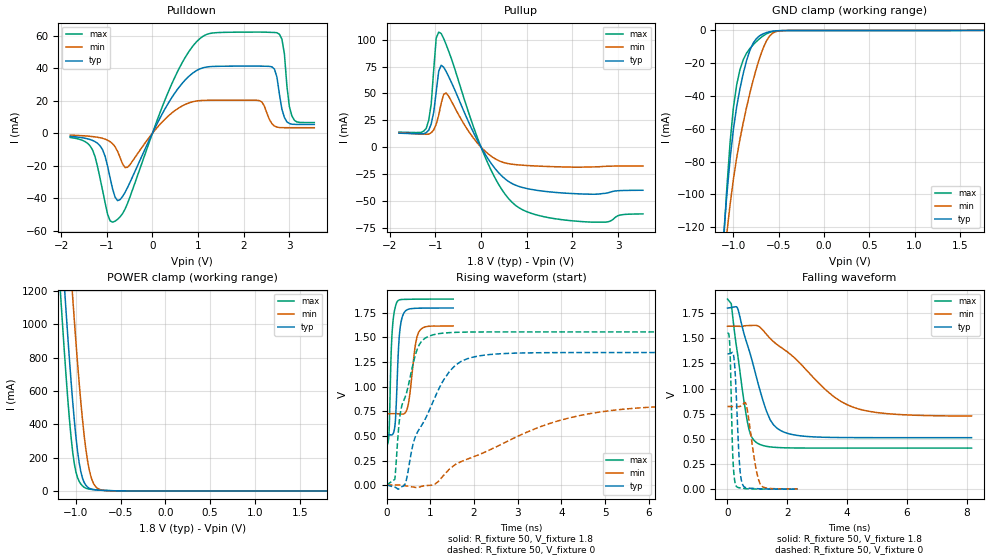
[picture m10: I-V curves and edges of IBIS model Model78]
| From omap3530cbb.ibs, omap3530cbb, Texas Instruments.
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| Model based on original model for BQ0234CS_7LM
|   Sub model BQ0234CS_7LM_PU_ON_1P8
[model]   Model78
|[Input Load]   PU
|[Output Drive]
|Voltage   1.8V
|Mode   I/O
Model_type   I/O
Polarity   Non-Inverting
Enable   Active-Low
Vinl =  0.63
Vinh =  1.17
Cref =  15.0000pF
Rref =  100.0000M
Vref =  0V
Vmeas =  0.9
C_comp   0.8818576p   0.7571797p   1.039848p
[Model Spec]
Vinl   0.63   0.567   0.6615
Vinh   1.17   1.053   1.2285
[Temperature Range]   25   125   -40
[Voltage Range]   1.8   1.62   1.89
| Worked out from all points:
|   slope of the pulldown table from 0 to 0.27 V, typ, clamps not added: 18.2 ohm
|   slope of the pullup table from 0 to 0.27 V, typ, clamps not added: 15.1 ohm
|   GND clamp passes 1 mA (typ) near -0.61 V on its own axis
|   POWER clamp passes 1 mA (typ) near -0.57 V on its own axis
|   rising waveform, R_fixture 50, V_fixture 1.8: 20-80 % time 81.1ps typ, 139ps min, 64.6ps max; typ from 0.513 V to 1.8 V
|   rising waveform, R_fixture 50, V_fixture 0: 20-80 % time 778ps typ, 2.51ns min, 382ps max; typ from 0.001 V to 1.35 V
|   falling waveform, R_fixture 50, V_fixture 1.8: 20-80 % time 757ps typ, 1.98ns min, 422ps max; typ from 1.8 V to 0.513 V
|   falling waveform, R_fixture 50, V_fixture 0: 20-80 % time 126ps typ, 250ps min, 81.5ps max; typ from 1.35 V to 0.002 V
[POWER_clamp]
-1.8V     7.03A      7.477A     6.772A
-1.182V   1.672A     2.34A      1.267A
-1.164V   1.518A     2.189A     1.114A
-1.127V   1.216A     1.889A     820.5mA
-1.073V   791.2mA    1.448A     431.2mA
-1.036V   538.2mA    1.164A     234.6mA
-963.6mV  169mA      647.7mA    57.34mA
-909.1mV  52.04mA    338.7mA    22.18mA
-872.7mV  24.24mA    189.9mA    13.43mA
-818.2mV  9.923mA    62.63mA    8.573mA
-709.1mV  3.896mA    5.034mA    3.819mA
1.8V      4.52nA     3.063nA    7.567nA
[Pulldown]
-1.8V     -1.896mA   -1.14mA    -2.549mA
-1.364V   -3.858mA   -1.868mA   -7.811mA
-1.145V   -7.758mA   -2.749mA   -27.9mA
-818.2mV  -39.37mA   -8.281mA   -54.21mA
-545.5mV  -33.5mA    -20.95mA   -43.25mA
654.5mV   30.89mA    16.9mA     43.69mA
1.418V    41.32mA    20.41mA    62.11mA
2.345V    41.43mA    20.12mA    62.44mA
2.618V    40.99mA    5.968mA    62.24mA
2.782V    24.07mA    3.525mA    61.09mA
3.055V    5.586mA    3.449mA    10.68mA
3.545V    5.467mA    3.446mA    6.63mA
[Pullup]
-1.8V     13mA       13.47mA    13.94mA
-1.2V     13.58mA    11.97mA    17.52mA
-1.091V   21.69mA    13.4mA     40.45mA
-1.036V   32.56mA    16.02mA    72.07mA
-981.8mV  51.55mA    21.35mA    101.5mA
-927.3mV  70.65mA    29.73mA    107.1mA
-818.2mV  74.4mA     49.19mA    101mA
-763.6mV  70.3mA     50.34mA    95.36mA
54.55mV   -4.056mA   -2.362mA   -5.695mA
709.1mV   -34.52mA   -16.04mA   -52.48mA
2.127V    -43.43mA   -18.65mA   -69.01mA
3.545V    -40.12mA   -17.52mA   -62.13mA
[GND_clamp]
-1.8V     -750.7mA   -623.3mA   -941.3mA
-1.109V   -125.7mA   -143.5mA   -129.9mA
-1.073V   -100.4mA   -123.9mA   -96.49mA
-1.036V   -78.3mA    -106.2mA   -68.25mA
-1V       -60.36mA   -90.76mA   -47.12mA
-963.6mV  -46.51mA   -77.61mA   -33.16mA
-890.9mV  -26.17mA   -56.18mA   -17.83mA
-818.2mV  -12.2mA    -38.34mA   -11.05mA
-709.1mV  -3.258mA   -16.62mA   -4.997mA
-600mV    -826.6uA   -3.389mA   -1.229mA
-490.9mV  -188uA     -312.2uA   -227.9uA
1.764V    -5.54uA    14.06uA    -26.2uA
[Ramp]
dV/dt_f  0.7805925/0.7635266n   0.541621/2.009354n   0.9011166/0.4265579n
dV/dt_r  0.8331727/0.7791177n  0.5087152/2.536557n   0.9651874/0.3825811n
R_load = 50
[Rising Waveform]
R_fixture = 50
V_fixture = 1.8
V_fixture_min = 1.62
V_fixture_max = 1.89
0s        513.1mV    725.9mV    409.7mV
54ps      513.1mV    725.9mV    525.7mV
130ps     512.5mV    726.3mV    1.582V
194ps     622.9mV    726.6mV    1.802V
228ps     912.4mV    726mV      1.853V
292ps     1.527V     723.4mV    1.881V
402ps     1.754V     725.8mV    1.887V
494ps     1.786V     818mV      1.887V
732ps     1.797V     1.553V     1.889V
1.522ns   1.799V     1.617V     1.89V
[Rising Waveform]
R_fixture = 50
V_fixture = 0
V_fixture_min = 0
V_fixture_max = 0
0s        1.238mV    776.6uV    1.504mV
188ps     -20.65mV   970uV      59.8mV
292ps     -33.42mV   1.059mV    659.3mV
416ps     6.516mV    -4.81mV    885.8mV
714ps     545.9mV    -24.04mV   1.396V
996ps     780mV      -2.038mV   1.517V
1.576ns   1.219V     211.3mV    1.552V
2.236ns   1.32V      332.8mV    1.556V
4.912ns   1.347V     744.7mV    1.556V
9.702ns   1.347V     819.9mV    1.556V
[Falling Waveform]
R_fixture = 50
V_fixture = 1.8
V_fixture_min = 1.62
V_fixture_max = 1.89
0s        1.8V       1.62V      1.89V
126ps     1.806V     1.62V      1.844V
340ps     1.797V     1.62V      1.338V
706ps     1.398V     1.627V     612.1mV
1.008ns   1.069V     1.625V     457.3mV
1.424ns   692.4mV    1.5V       421.6mV
2.118ns   547.2mV    1.338V     411.3mV
3.388ns   516.2mV    961.3mV    409.7mV
4.186ns   513.8mV    817.3mV    409.7mV
8.16ns    513.1mV    729.2mV    409.7mV
[Falling Waveform]
R_fixture = 50
V_fixture = 0
V_fixture_min = 0
V_fixture_max = 0
0s        1.347V     823.1mV    1.556V
76ps      1.347V     823.1mV    1.438V
178ps     1.358V     822.4mV    327.4mV
276ps     1.051V     821.8mV    41.08mV
396ps     278.2mV    822.6mV    15.58mV
512ps     43.24mV    841.3mV    11.19mV
628ps     15.33mV    841.4mV    5.916mV
946ps     7.471mV    216.6mV    3.252mV
1.09ns    5.066mV    54.83mV    2.793mV
2.348ns   1.936mV    4.026mV    1.594mV
